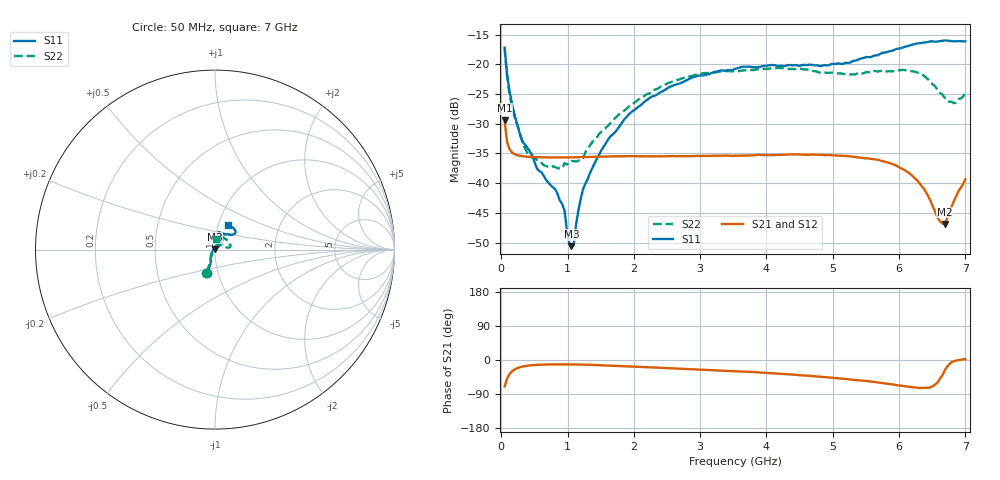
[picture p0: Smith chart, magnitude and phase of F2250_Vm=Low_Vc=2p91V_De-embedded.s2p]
! Integrated Device Technology
! Corporate Headquarters
! 6024 Silver Creek Valley Road
! San Jose, CA 95138  USA
! Phone:  1-408-284-8200
! Toll Free:  1-800-223-1366
! Webpage:  http://www.idt.com/
! Timing and RF Division
! 515 Groton Road, Suite 102
! Westford, MA 01886-6024
! Device:  F2250
! Description: Voltage Variable RF Attenuator
! Frequency:  50.0 -  6000.00 MHz
! Package:  3x3 mm Thin QFN Plastic Package: 16 pin
! Ports:  2 RF, 3 DC
!  Pin  1  = GND
!  Pin  2  = NC
!  Pin  3  = RF1  = Port 1
!  Pin  4  = NC
!  Pin  5  = GND
!  Pin  6  = GND
!  Pin  7  = GND
!  Pin  8  = GND
!  Pin  9  = NC
!  Pin 10  = RF2  = Port 2
!  Pin 11  = NC
!  Pin 12  = GND
!  Pin 13  = GND
!  Pin 14  = VCNTRL
!  Pin 15  = VDD
!  Pin 16  = VMODE
! Vcntrl:  2.910 Volts
! Vmode:  +0.000 Volts
! Vdd:  +3.30  Volts
! Current:  1.177 mA
! Data:  The device was measured on a the F2250 evaluation board which has
!  individual transmission lines to the RF pins.  Data was collected
!  using a calibrated network analyzer.  The evaluation board was
!  de-embedded using a TRL calibration technique.
!  The reference plane is the edge of the package pin.
! Misc:  SN 10
!  Action Tracker AT0258
! Date Measured:  2014-11-26
! Date:  2015-10-15  MJV
! Note:
!  Integrated Device Technology supplies this data as a sample of measured
!  data at the package pin for this product.  Your particular data for this
!  product may vary.
!  Data was taken at 25 degrees C.
!  Integrated Device Technology reserves the right to change this data at anytime.
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# GHz S dB R 50
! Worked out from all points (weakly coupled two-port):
!   201 points, 50 MHz to 7 GHz, reference 50 ohm
!   highest |S21| = -29.41 dB at 50 MHz (marker M1); lowest = -46.9 dB at 6.687 GHz (marker M2)
!   lowest |S11| = -50.6 dB at 1.058 GHz (marker M3), VSWR 1.01, Z = 49.8 + j0.246 ohm
!   |S11| at or under -10 dB: start of sweep to end of sweep
!   |S22| runs from -37.5 to -17.3 dB; largest |S21 - S12| = 6.2e-05
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0.05  -17.18 -108.7  -29.41 -69.8  -29.41 -69.8  -17.28 -111.0
0.08475  -21.45 -107.5  -32.92 -50.3  -32.92 -50.3  -21.74 -110.2
0.15425  -26.24 -116.6  -34.76 -31.2  -34.76 -31.1  -26.81 -122.5
0.29325  -32.22 -127.9  -35.43 -18.5  -35.43 -18.5  -32.09 -137.4
0.3975  -34.10 -141.9  -35.56 -15.0  -35.56 -15.0  -35.05 -160.4
0.91875  -43.52 157.7  -35.69 -11.5  -35.68 -11.5  -37.55 133.4
0.9535  -44.61 170.1  -35.69 -11.5  -35.68 -11.5  -36.64 131.0
1.023  -50.05 143.7  -35.68 -11.6  -35.67 -11.6  -36.63 115.9
1.05775  -50.61 123.2  -35.67 -11.7  -35.66 -11.6  -36.29 110.7
1.0925  -50.48 89.6  -35.66 -11.7  -35.66 -11.7  -36.31 106.3
1.162  -44.65 56.9  -35.64 -11.9  -35.64 -11.9  -36.21 95.5
1.2315  -41.07 44.2  -35.61 -12.1  -35.61 -12.1  -35.79 85.7
1.6485  -32.11 42.0  -35.52 -14.6  -35.52 -14.7  -29.87 64.6
1.96125  -28.05 42.2  -35.46 -17.2  -35.46 -17.2  -26.81 56.8
2.37825  -24.87 47.3  -35.48 -20.3  -35.48 -20.3  -23.99 56.8
3.525  -20.79 72.5  -35.40 -29.5  -35.40 -29.6  -21.19 74.7
4.7065  -20.17 72.3  -35.19 -42.6  -35.19 -42.6  -21.14 72.2
5.85325  -17.81 40.4  -36.63 -63.4  -36.63 -63.5  -21.14 23.1
6.27025  -16.51 40.0  -39.50 -72.9  -39.51 -72.9  -21.37 9.7
6.68725  -15.99 48.7  -46.90 -27.6  -46.87 -27.5  -25.63 28.6
6.861  -16.13 55.1  -42.21 -1.3  -42.17 -1.4  -26.45 57.9
7  -16.13 63.2  -39.36 1.9  -39.33 1.7  -24.63 83.0
